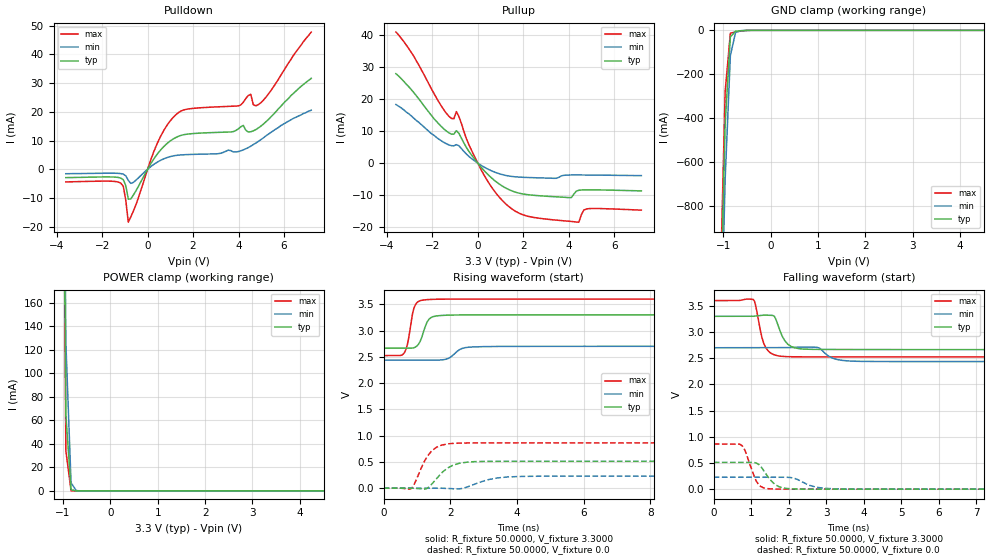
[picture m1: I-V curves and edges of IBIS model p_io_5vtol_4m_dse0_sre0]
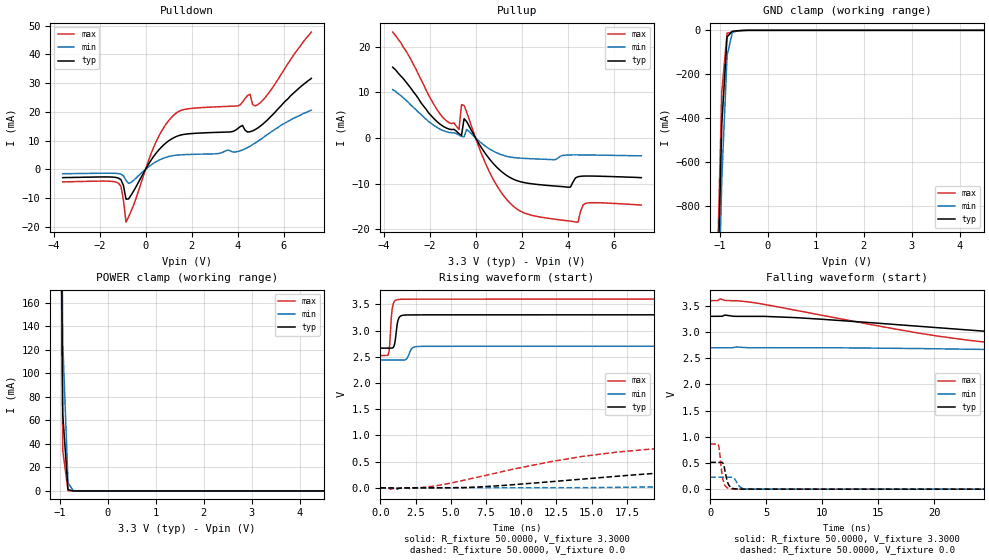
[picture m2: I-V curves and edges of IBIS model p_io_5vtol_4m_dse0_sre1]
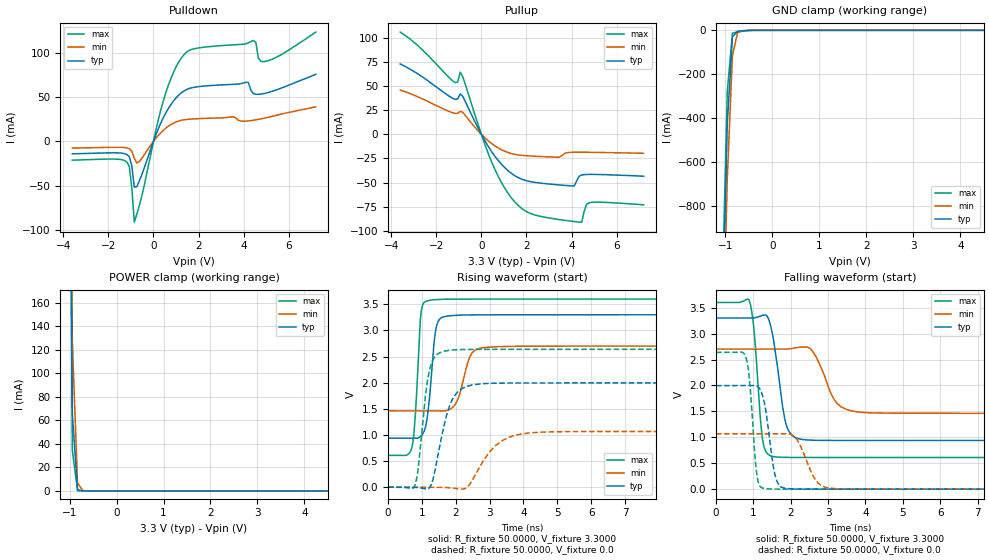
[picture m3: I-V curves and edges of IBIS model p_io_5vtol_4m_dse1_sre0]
| IBIS file nevis_80lqfp_normal.ibs generated by Daphne version: 2018.03.27
[IBIS Ver]   5.0
[Comment Char]   |_char
[File Name]   nevis_80lqfp_normal.ibs
[File Rev]   1
[Date]   Tue Nov  6 16:55:37 2018
[Source]   NXP Viper 2018.03.27
[Notes]
[Disclaimer] IMPORTANT NOTICE
  This information is provided on an AS IS basis and without warranty.
  IN NO EVENT SHALL NXP BE LIABLE FOR INCIDENTAL OR CONSEQUENTIAL
  DAMAGES ARISING FROM USE OF THIS INFORMATION. THIS DISCLAIMER OF
  WARRANTY EXTENDS TO THE USER OF THE INFORMATION, AND TO THEIR CUSTOMERS
  OR USERS OF PRODUCTS  AND IS IN LIEU OF ALL WARRANTIES WHETHER EXPRESS,
  IMPLIED, OR STATUTORY, INCLUDING IMPLIED WARRANTIES OF MERCHANTABILITY
  OR FITNESS FOR PARTICULAR PURPOSE.
  NXP does not represent or warrant that the information furnished
  hereunder is free of infringement of any third party patents,
  copyrights, trade secrets, or other intellectual property rights.
  NXP does not represent or warrant that the information is free of
  defect, or that it meets any particular standard, requirements or need
  of the user of the infomation or their customers.
  NXP reserves the right to change the information in this file
  without notice.
   http://www.nxp.com
[Copyright]   (C) Copyright NXP 2004 - 2018, All Rights Reserved.
|   NEVIS:80LQFP
[Component]   NEVIS:80LQFP
[Manufacturer]   NXP
[Package]
| variable   typ   min   max
R_pkg   0.14792   0.086913   0.16418
L_pkg   3.915e-09   3.208e-09   4.513e-09
C_pkg   6.180e-13   5.453e-13   7.626e-13
[Pin] signal_name   model_name   R_pin   L_pin   C_pin
1   TCK   p_io_5vtol_4m   0.1569   4.463e-09 6.104e-13
2   RESETB   p_vpp_5vtol_4m   0.086913  3.716e-09 7.626e-13
3   GPIOC0   p_io_5vtol_4m   0.1464   4.224e-09 6.498e-13
4   GPIOC1   p_io_5vtol_4m   0.14132   4.089e-09 6.578e-13
5   GPIOC2   p_io_5vtol_4m   0.13836   3.977e-09 6.265e-13
6   GPIOF8   p_io_5vtol_4m   0.13627   3.873e-09 6.056e-13
7   GPIOD6   p_io_5vtol_4m   0.13889   3.853e-09 6.753e-13
8   GPIOD5   p_io_5vtol_4m   0.13733   3.661e-09 5.770e-13
9   GPIOC3   p_io_5vtol_4m   0.13967   3.625e-09 5.687e-13
10   GPIOC4   p_io_5vtol_4m   0.14324   3.260e-09 5.584e-13
11   VSS   GND   NA   NA   NA
12   VDD   POWER   NA   NA   NA
13   GPIOA7   p_io_5vtol_4m   0.14268   3.208e-09 5.596e-13
14   GPIOA6   p_io_5vtol_4m   0.13768   3.627e-09 5.771e-13
15   GPIOA5   p_io_5vtol_4m   0.13834   3.794e-09 6.092e-13
16   GPIOA4   p_io_5vtol_4m   0.14103   3.970e-09 6.163e-13
17   GPIOA0   p_io_5vtol_4m   0.14398   4.103e-09 6.334e-13
18   GPIOA1   p_io_5vtol_4m   0.14886   4.265e-09 6.523e-13
19   GPIOA2   p_io_5vtol_4m   0.15426   4.392e-09 6.811e-13
20   GPIOA3   p_io_5vtol_4m   0.15897   4.513e-09 6.239e-13
21   GPIOB7   p_io_5vtol_4m   0.16119   4.455e-09 6.055e-13
22   GPIOC5   p_io_5vtol_4m   0.089097  3.705e-09 7.594e-13
23   GPIOB6   p_io_5vtol_4m   0.15247   4.133e-09 6.437e-13
24   GPIOB5   p_io_5vtol_4m   0.15127   3.904e-09 6.550e-13
25   GPIOB4   p_io_5vtol_4m   0.15683   3.445e-09 6.248e-13
26   VDDA   POWER   NA   NA   NA
27   VSSA   GND   NA   NA   NA
28   GPIOB0   p_io_5vtol_4m   0.15671   3.227e-09 5.981e-13
29   GPIOB1   p_io_5vtol_4m   0.16081   3.366e-09 5.864e-13
30   VDD   POWER   NA   NA   NA
31   GPIOB2   p_io_5vtol_4m   0.16418   3.339e-09 5.839e-13
32   GPIOA11   p_io_5vtol_4m   0.15928   3.765e-09 5.648e-13
33   GPIOB8   p_io_5vtol_4m   0.15865   3.789e-09 5.728e-13
34   GPIOB3   p_io_5vtol_4m   0.15776   3.412e-09 5.725e-13
35   VDD33   POWER   NA   NA   NA
36   VSS   GND   NA   NA   NA
37   GPIOD7   p_io_5vtol_4m   0.15661   3.718e-09 6.186e-13
38   GPIOG11   p_io_5vtol_4m   0.15508   4.092e-09 6.428e-13
39   GPIOC6   p_io_5vtol_4m   0.15749   4.282e-09 6.708e-13
40   GPIOC7   p_io_5vtol_4m   0.16015   4.420e-09 6.086e-13
41   GPIOC8   p_io_5vtol_4m   0.155   4.392e-09 6.129e-13
42   GPIOC9   p_io_5vtol_4m   0.15023   4.314e-09 6.746e-13
43   GPIOC10   p_io_5vtol_4m   0.14475   4.157e-09 6.325e-13
44   GPIOF0   p_io_5vtol_4m   0.14034   4.038e-09 6.186e-13
45   GPIOF10   p_io_5vtol_4m   0.13729   3.935e-09 5.995e-13
46   GPIOF9   p_io_5vtol_4m   0.13506   3.812e-09 5.800e-13
47   GPIOC11   p_io_5vtol_4m   0.13569   3.773e-09 5.736e-13
48   GPIOC12   p_io_5vtol_4m   0.13431   3.631e-09 5.670e-13
49   GPIOF2   p_io_5vtol_4m   0.13671   3.678e-09 5.521e-13
50   GPIOF3   p_io_5vtol_4m   0.13715   3.575e-09 5.842e-13
51   GPIOF4   p_io_5vtol_4m   0.13922   3.499e-09 5.749e-13
52   GPIOF5   p_io_5vtol_4m   0.14513   3.371e-09 5.453e-13
53   VSS   GND   NA   NA   NA
54   VDD33   POWER   NA   NA   NA
55   GPIOE0   p_io_5vtol_4m   0.14382   3.257e-09 5.801e-13
56   GPIOE1   p_io_5vtol_4m   0.14278   3.728e-09 6.043e-13
57   GPIOG2   p_io_5vtol_4m   0.14594   4.015e-09 5.873e-13
58   GPIOG3   p_io_5vtol_4m   NA   NA   NA
59   GPIOE2   p_io_5vtol_4m   0.15025   4.275e-09 6.580e-13
60   GPIOE3   p_io_5vtol_4m   0.15495   4.361e-09 6.103e-13
61   GPIOC13   p_io_5vtol_4m   0.15782   4.510e-09 6.206e-13
62   GPIOF1   p_io_5vtol_4m   0.15552   4.467e-09 6.836e-13
63   GPIOG0   p_io_5vtol_4m   0.15239   4.349e-09 6.443e-13
64   GPIOG1   p_io_5vtol_4m   0.15   4.246e-09 6.251e-13
65   GPIOE4   p_io_5vtol_4m   0.15123   4.216e-09 6.160e-13
66   GPIOE5   p_io_5vtol_4m   0.14973   4.115e-09 6.183e-13
67   GPIOE6   p_io_5vtol_4m   0.1495   4.063e-09 6.138e-13
68   GPIOE7   p_io_5vtol_4m   0.14975   3.950e-09 6.053e-13
69   GPIOG6   p_io_5vtol_4m   0.15342   4.029e-09 5.810e-13
70   GPIOC14   p_io_5vtol_4m   0.15484   3.948e-09 6.094e-13
71   GPIOC15   p_io_5vtol_4m   0.15791   3.901e-09 6.007e-13
72   GPIOG7   p_io_5vtol_4m   0.16357   3.560e-09 5.812e-13
73   VDD   POWER   NA   NA   NA
74   GPIOF6   p_io_5vtol_4m   0.16081   3.496e-09 6.833e-13
75   GPIOF7   p_io_5vtol_4m   0.16138   3.528e-09 6.113e-13
76   VDD33   POWER   NA   NA   NA
77   VSS   GND   NA   NA   NA
78   TDO   p_io_5vtol_4m   0.16287   3.741e-09 6.499e-13
79   TMS   p_io_5vtol_4m   0.16067   4.282e-09 7.221e-13
80   TDI   p_io_5vtol_4m   0.16215   4.444e-09 6.324e-13
81   NC   NC   NA   NA   NA
[Pin Mapping]   pulldown_ref   pullup_ref
1   NC   NC
2   NC   NC
3   NC   NC
4   NC   NC
5   NC   NC
6   NC   NC
7   NC   NC
8   NC   NC
9   NC   NC
10   NC   NC
11   VSS   NC
12   NC   VDD
13   NC   NC
14   NC   NC
15   NC   NC
16   NC   NC
17   NC   NC
18   NC   NC
19   NC   NC
20   NC   NC
21   NC   NC
22   NC   NC
23   NC   NC
24   NC   NC
25   NC   NC
26   NC   VDDA
27   VSSA   NC
28   NC   NC
29   NC   NC
30   NC   VDD
31   NC   NC
32   NC   NC
33   NC   NC
34   NC   NC
35   NC   VDD33
36   VSS   NC
37   NC   NC
38   NC   NC
39   NC   NC
40   NC   NC
41   NC   NC
42   NC   NC
43   NC   NC
44   NC   NC
45   NC   NC
46   NC   NC
47   NC   NC
48   NC   NC
49   NC   NC
50   NC   NC
51   NC   NC
52   NC   NC
53   VSS   NC
54   NC   VDD33
55   NC   NC
56   NC   NC
57   NC   NC
58   NC   NC
59   NC   NC
60   NC   NC
61   NC   NC
62   NC   NC
63   NC   NC
64   NC   NC
65   NC   NC
66   NC   NC
67   NC   NC
68   NC   NC
69   NC   NC
70   NC   NC
71   NC   NC
72   NC   NC
73   NC   VDD
74   NC   NC
75   NC   NC
76   NC   VDD33
77   VSS   NC
78   NC   NC
79   NC   NC
80   NC   NC
81   NC   NC
|*   Model Selector   *
[Model Selector] p_io_5vtol_4m
p_io_5vtol_4m_dse1_sre0   io, full drive mode without slew rate
p_io_5vtol_4m_dse1_sre1   io, full drive mode with slew rate
p_io_5vtol_4m_dse0_sre0   io, low drive mode without slew rate
p_io_5vtol_4m_dse0_sre1   io, low drive mode with slew rate
| End [Component] NEVIS:80LQFP
| Models and submodels in the file (5): p_io_5vtol_4m_dse0_sre0 (I/O), p_io_5vtol_4m_dse0_sre1 (I/O), p_io_5vtol_4m_dse1_sre0 (I/O), p_io_5vtol_4m_dse1_sre1 (I/O), p_vpp_5vtol_4m (I/O_open_drain)
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[Model] p_io_5vtol_4m_dse0_sre0
|   Model p_io_5vtol_4m_dse0_sre0
| Library cells for typ/min/max conditions are connected as defined below:
|  pad - External Pad
|  ipp_do - Core Input
|  ipp_obe - Output Buffer Enable
|  esd_boost - vdd_s_3v
|  esd_bus - vdd_s_3v
|  ipp_ame - vss_s_lv
|  ipp_dse - vss_s_lv
|  ipp_ina40a_5vtol - NC
|  ipp_ina40b_5vtol - NC
|  ipp_ina_5vtol - NC
|  ipp_ina_mux_3v - NC
|  ipp_ind - NC
|  ipp_ind_3v - NC
|  ipp_pue - vss_s_lv
|  ipp_sre - vss_s_lv
|  tie_3v - vdd_s_3v
|  tie_hi - vdd_s_lv
|  vbuf_3v - vdd_s_3v
|  vdd_bulk_lv - vdd_s_lv
|  vdd_s_3v - vdd_s_3v
|  vdd_s_lv - vdd_s_lv
|  vss_bulk - vss_s_3v
|  vss_s_3v - vss_s_3v
|  vss_s_lv - vss_s_lv
| All other pins connected to ground
Model_type I/O
Polarity   Non-Inverting
Enable   Active-High
Vinl =   1.1550V
Vinh =   2.3100V
Vmeas =  1.6500V
Cref =   25.0000pF
Rref =   0.5000k
Vref =   0.0V
C_comp   2.7442pF   2.6088pF   2.9166pF
[Temperature Range]   25.0000   0.1250k   -40.0000
[Voltage Range]   3.3000V   2.7000V   3.6000V
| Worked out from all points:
|   slope of the pulldown table from 0 to 0.495 V, typ, clamps not added: 82.8 ohm
|   slope of the pullup table from 0 to 0.495 V, typ, clamps not added: 127 ohm
|   GND clamp passes 1 mA (typ) near -0.56 V on its own axis
|   POWER clamp passes 1 mA (typ) near -0.82 V on its own axis
|   rising waveform, R_fixture 50.0000, V_fixture 3.3000: 20-80 % time 220ps typ, 318ps min, 177ps max; typ from 2.66 V to 3.3 V
|   rising waveform, R_fixture 50.0000, V_fixture 0.0: 20-80 % time 520ps typ, 708ps min, 427ps max; typ from 0 V to 0.512 V
|   falling waveform, R_fixture 50.0000, V_fixture 3.3000: 20-80 % time 253ps typ, 333ps min, 210ps max; typ from 3.3 V to 2.66 V
|   falling waveform, R_fixture 50.0000, V_fixture 0.0: 20-80 % time 337ps typ, 455ps min, 264ps max; typ from 0.512 V to 0 V
[Pulldown]
|Voltage   I(typ)   I(min)   I(max)
-3.6V     -2.92mA    -1.56mA    -4.41mA
-1.18V    -3.075mA   -1.514mA   -4.85mA
-1.07V    -3.642mA   -1.711mA   -5.917mA
-850mV    -10.41mA   -3.881mA   -18.45mA
360mV     4.579mA    2.156mA    7.833mA
1.13V     10.56mA    4.658mA    18.11mA
1.79V     12.28mA    5.123mA    21mA
3.99V     14.08mA    6.16mA     22.06mA
4.54V     13.07mA    8.03mA     26.11mA
4.65V     13.38mA    8.6mA      22.52mA
4.87V     14.37mA    9.7mA      22.49mA
7.2V      31.7mA     20.6mA     47.8mA
[Pullup]
|Voltage   I(typ)   I(min)   I(max)
-3.6V     27.9mA     18.3mA     40.9mA
-2.81V    22mA       14mA       33.3mA
-1.38V    10.01mA    6.04mA     15.54mA
-1.05V    9.045mA    5.403mA    13.85mA
-940mV    10.12mA    5.768mA    16.08mA
-390mV    3.678mA    2.088mA    5.744mA
270mV     -2.258mA   -1.197mA   -3.638mA
1.48V     -8.613mA   -4.152mA   -14.19mA
4.01V     -10.78mA   -3.728mA   -18.16mA
4.45V     -8.487mA   -3.709mA   -18.45mA
4.78V     -8.342mA   -3.73mA    -14.33mA
7.2V      -8.69mA    -3.91mA    -14.69mA
[GND_clamp]
|Voltage   I(typ)   I(min)   I(max)
-3.6V     -31.15A    -31.13A    -31.21A
-1.07V    -1.387A    -1.641A    -1.238A
-960mV    -429.3mA   -680.2mA   -281.1mA
-850mV    -29.75mA   -116.1mA   -13.24mA
-740mV    -4.234mA   -9.703mA   -7.092mA
-630mV    -1.925mA   -1.63mA    -3.569mA
-410mV    -31.96uA   -64.36uA   -35uA
7.2V      0A         0A         0A
[POWER_clamp]
|Voltage   I(typ)   I(min)   I(max)
-3.6V     31.35A     31.03A     31.61A
-1.05V    682.2mA    740.4mA    662.9mA
-940mV    65.1mA     126.6mA    34.32mA
-830mV    1.105mA    6.829mA    165.4uA
-720mV    15.33uA    281.3uA    694.4nA
-610mV    212.1nA    11.41uA    2.964nA
7.2V      0A         0A         0A
[Ramp]
| variable   typ   min   max
dV/dt_r  0.3070/0.5203n   0.1368/0.7078n   0.5174/0.4265n
dV/dt_f  0.3816/0.2526n   0.1581/0.3329n   0.6454/0.2102n
R_load = 50.0000
[Rising Waveform]
R_fixture= 50.0000
V_fixture= 3.3000
V_fixture_min= 2.7000
V_fixture_max= 3.6000
|time   V(typ)   V(min)   V(max)
0s        2.664V     2.436V     2.524V
610.3ps   2.664V     2.436V     2.569V
714.5ps   2.664V     2.436V     2.741V
910.9ps   2.675V     2.436V     3.431V
1.094ns   2.792V     2.437V     3.568V
1.273ns   3.119V     2.437V     3.588V
1.552ns   3.276V     2.437V     3.596V
2.35ns    3.298V     2.659V     3.599V
2.979ns   3.3V       2.694V     3.599V
20ns      3.3V       2.7V       3.6V
[Rising Waveform]
R_fixture= 50.0000
V_fixture= 0.0
V_fixture_min= 0.0
V_fixture_max= 0.0
|time   V(typ)   V(min)   V(max)
0s        1.096nV    96.66nV    914.3pV
817.3ps   -174.2uV   1.791uV    -11.85mV
1.238ns   -20.09mV   132uV      527.3mV
1.432ns   68.46mV    364.3uV    703.1mV
1.774ns   310.6mV    -2.683mV   823mV
2.042ns   424.3mV    -10.1mV    850.1mV
2.694ns   503.4mV    66.34mV    860.8mV
3.192ns   509.9mV    168.5mV    861.5mV
4.049ns   511.3mV    221.6mV    861.7mV
20ns      511.7mV    228.1mV    862.3mV
[Falling Waveform]
R_fixture= 50.0000
V_fixture= 3.3000
V_fixture_min= 2.7000
V_fixture_max= 3.6000
|time   V(typ)   V(min)   V(max)
0s        3.3V       2.7V       3.6V
1.056ns   3.301V     2.7V       3.62V
1.285ns   3.321V     2.7V       2.894V
1.39ns    3.322V     2.7V       2.695V
1.614ns   3.301V     2.7V       2.565V
1.898ns   2.83V      2.7V       2.531V
2.744ns   2.668V     2.71V      2.525V
3.178ns   2.667V     2.499V     2.525V
3.812ns   2.665V     2.441V     2.525V
20ns      2.664V     2.436V     2.524V
[Falling Waveform]
R_fixture= 50.0000
V_fixture= 0.0
V_fixture_min= 0.0
V_fixture_max= 0.0
|time   V(typ)   V(min)   V(max)
0s        511.8mV    228.1mV    862.4mV
740.7ps   511.8mV    228.1mV    838mV
824.6ps   511.7mV    228.1mV    750.7mV
1.166ns   486.7mV    228.1mV    119mV
1.481ns   202.1mV    228.1mV    6.302mV
1.652ns   81.2mV     228mV      2.01mV
1.911ns   16.02mV    227.7mV    767.9uV
2.752ns   448uV      36.41mV    432.9uV
3.473ns   288.4uV    2.353mV    359uV
20ns      60.38uV    38.43uV    87.29uV
[Model] p_io_5vtol_4m_dse0_sre1
|   Model p_io_5vtol_4m_dse0_sre1
| Library cells for typ/min/max conditions are connected as defined below:
|  pad - External Pad
|  ipp_do - Core Input
|  ipp_obe - Output Buffer Enable
|  esd_boost - vdd_s_3v
|  esd_bus - vdd_s_3v
|  ipp_ame - vss_s_lv
|  ipp_dse - vss_s_lv
|  ipp_ina40a_5vtol - NC
|  ipp_ina40b_5vtol - NC
|  ipp_ina_5vtol - NC
|  ipp_ina_mux_3v - NC
|  ipp_ind - NC
|  ipp_ind_3v - NC
|  ipp_pue - vss_s_lv
|  ipp_sre - vdd_s_lv
|  tie_3v - vdd_s_3v
|  tie_hi - vdd_s_lv
|  vbuf_3v - vdd_s_3v
|  vdd_bulk_lv - vdd_s_lv
|  vdd_s_3v - vdd_s_3v
|  vdd_s_lv - vdd_s_lv
|  vss_bulk - vss_s_3v
|  vss_s_3v - vss_s_3v
|  vss_s_lv - vss_s_lv
| All other pins connected to ground
Model_type I/O
Polarity   Non-Inverting
Enable   Active-High
Vinl =   1.1550V
Vinh =   2.3100V
Vmeas =  1.6500V
Cref =   25.0000pF
Rref =   0.5000k
Vref =   0.0V
C_comp   2.7442pF   2.6088pF   2.9166pF
[Temperature Range]   25.0000   0.1250k   -40.0000
[Voltage Range]   3.3000V   2.7000V   3.6000V
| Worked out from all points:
|   slope of the pulldown table from 0 to 0.495 V, typ, clamps not added: 82.8 ohm
|   slope of the pullup table from 0 to 0.495 V, typ, clamps not added: 127 ohm
|   GND clamp passes 1 mA (typ) near -0.56 V on its own axis
|   POWER clamp passes 1 mA (typ) near -0.82 V on its own axis
|   rising waveform, R_fixture 50.0000, V_fixture 3.3000: 20-80 % time 192ps typ, 268ps min, 163ps max; typ from 2.66 V to 3.3 V
|   rising waveform, R_fixture 50.0000, V_fixture 0.0: 20-80 % time 17.3ns typ, 32.4ns min, 10.8ns max; typ from 0 V to 0.512 V
|   falling waveform, R_fixture 50.0000, V_fixture 3.3000: 20-80 % time 29.9ns typ, 51ns min, 19.5ns max; typ from 3.3 V to 2.66 V
|   falling waveform, R_fixture 50.0000, V_fixture 0.0: 20-80 % time 342ps typ, 422ps min, 300ps max; typ from 0.512 V to 0 V
[Pulldown]
|Voltage   I(typ)   I(min)   I(max)
-3.6V     -2.92mA    -1.56mA    -4.41mA
-1.18V    -3.075mA   -1.514mA   -4.85mA
-1.07V    -3.642mA   -1.711mA   -5.917mA
-850mV    -10.41mA   -3.881mA   -18.45mA
360mV     4.579mA    2.156mA    7.833mA
1.13V     10.56mA    4.658mA    18.11mA
1.79V     12.28mA    5.123mA    21mA
3.99V     14.08mA    6.16mA     22.06mA
4.54V     13.07mA    8.03mA     26.11mA
4.65V     13.38mA    8.6mA      22.52mA
4.87V     14.37mA    9.7mA      22.49mA
7.2V      31.7mA     20.6mA     47.8mA
[Pullup]
|Voltage   I(typ)   I(min)   I(max)
-3.6V     15.5mA     10.6mA     23.2mA
-1.38V    2.47mA     1.56mA     4.28mA
-720mV    935.3uA    641.5uA    1.84mA
-610mV    580.7uA    348.6uA    7.293mA
-500mV    4.215mA    257.3uA    7.125mA
-390mV    3.605mA    1.85mA     5.718mA
710mV     -5.257mA   -2.715mA   -8.512mA
1.81V     -9.375mA   -4.366mA   -15.61mA
4.12V     -10.77mA   -3.714mA   -18.22mA
4.45V     -8.487mA   -3.709mA   -18.45mA
4.78V     -8.342mA   -3.73mA    -14.33mA
7.2V      -8.69mA    -3.91mA    -14.69mA
[GND_clamp]
|Voltage   I(typ)   I(min)   I(max)
-3.6V     -31.15A    -31.13A    -31.21A
-1.07V    -1.387A    -1.641A    -1.238A
-960mV    -429.3mA   -680.2mA   -281.1mA
-850mV    -29.75mA   -116.1mA   -13.24mA
-740mV    -4.234mA   -9.703mA   -7.092mA
-630mV    -1.925mA   -1.63mA    -3.569mA
-410mV    -31.96uA   -64.36uA   -35uA
7.2V      0A         0A         0A
[POWER_clamp]
|Voltage   I(typ)   I(min)   I(max)
-3.6V     31.35A     31.03A     31.61A
-1.05V    682.2mA    740.4mA    662.9mA
-940mV    65.1mA     126.6mA    34.32mA
-830mV    1.105mA    6.829mA    165.4uA
-720mV    15.33uA    281.3uA    694.4nA
-610mV    212.1nA    11.41uA    2.964nA
7.2V      0A         0A         0A
[Ramp]
| variable   typ   min   max
dV/dt_r  0.3071/17.2926n   0.1369/32.3674n   0.5175/10.7611n
dV/dt_f  0.3817/29.8719n   0.1576/51.0200n   0.6456/19.5314n
R_load = 50.0000
[Rising Waveform]
R_fixture= 50.0000
V_fixture= 3.3000
V_fixture_min= 2.7000
V_fixture_max= 3.6000
|time   V(typ)   V(min)   V(max)
0s        2.664V     2.437V     2.524V
605.3ps   2.664V     2.437V     2.579V
657.9ps   2.664V     2.437V     2.693V
807.7ps   2.664V     2.437V     3.325V
923.6ps   2.679V     2.436V     3.511V
1.276ns   3.209V     2.437V     3.592V
1.646ns   3.293V     2.437V     3.597V
2.341ns   3.298V     2.679V     3.598V
3.739ns   3.299V     2.699V     3.598V
250ns     3.3V       2.7V       3.6V
[Rising Waveform]
R_fixture= 50.0000
V_fixture= 0.0
V_fixture_min= 0.0
V_fixture_max= 0.0
|time   V(typ)   V(min)   V(max)
0s        1.096nV    96.66nV    914.3pV
730.2ps   540.1uV    1.417uV    -25.29mV
3.533ns   -267.8uV   -118.1uV   22.43mV
11.84ns   111.3mV    1.042mV    487mV
16.8ns    222mV      9.094mV    681.3mV
24.08ns   354mV      38.46mV    807.6mV
31.02ns   430.3mV    75.05mV    845.8mV
49.75ns   501.2mV    160.4mV    861.8mV
86.96ns   511.7mV    219.4mV    862.5mV
250ns     511.8mV    228.1mV    862.5mV
[Falling Waveform]
R_fixture= 50.0000
V_fixture= 3.3000
V_fixture_min= 2.7000
V_fixture_max= 3.6000
|time   V(typ)   V(min)   V(max)
0s        3.3V       2.7V       3.6V
896.8ps   3.3V       2.7V       3.63V
3.769ns   3.3V       2.7V       3.565V
18.49ns   3.112V     2.686V     2.984V
25.66ns   2.998V     2.664V     2.78V
33.75ns   2.887V     2.635V     2.66V
43.81ns   2.796V     2.595V     2.594V
65.21ns   2.714V     2.521V     2.543V
96.83ns   2.677V     2.472V     2.527V
250ns     2.664V     2.437V     2.524V
[Falling Waveform]
R_fixture= 50.0000
V_fixture= 0.0
V_fixture_min= 0.0
V_fixture_max= 0.0
|time   V(typ)   V(min)   V(max)
0s        511.8mV    228.1mV    862.4mV
711.3ps   511.8mV    228.1mV    851.3mV
813.8ps   511.8mV    228.1mV    743.1mV
1.045ns   511.3mV    228.1mV    281.6mV
1.18ns    474mV      228.1mV    137.9mV
1.57ns    116.7mV    228mV      19.01mV
2.147ns   7.963mV    204.4mV    2.261mV
2.747ns   1.249mV    29.86mV    1.357mV
3.983ns   641.3uV    486.1uV    1mV
250ns     26.94nV    927.1nV    8.795nV
[Model] p_io_5vtol_4m_dse1_sre0
|   Model p_io_5vtol_4m_dse1_sre0
| Library cells for typ/min/max conditions are connected as defined below:
|  pad - External Pad
|  ipp_do - Core Input
|  ipp_obe - Output Buffer Enable
|  esd_boost - vdd_s_3v
|  esd_bus - vdd_s_3v
|  ipp_ame - vss_s_lv
|  ipp_dse - vdd_s_lv
|  ipp_ina40a_5vtol - NC
|  ipp_ina40b_5vtol - NC
|  ipp_ina_5vtol - NC
|  ipp_ina_mux_3v - NC
|  ipp_ind - NC
|  ipp_ind_3v - NC
|  ipp_pue - vss_s_lv
|  ipp_sre - vss_s_lv
|  tie_3v - vdd_s_3v
|  tie_hi - vdd_s_lv
|  vbuf_3v - vdd_s_3v
|  vdd_bulk_lv - vdd_s_lv
|  vdd_s_3v - vdd_s_3v
|  vdd_s_lv - vdd_s_lv
|  vss_bulk - vss_s_3v
|  vss_s_3v - vss_s_3v
|  vss_s_lv - vss_s_lv
| All other pins connected to ground
Model_type I/O
Polarity   Non-Inverting
Enable   Active-High
Vinl =   1.1550V
Vinh =   2.3100V
Vmeas =  1.6500V
Cref =   25.0000pF
Rref =   0.5000k
Vref =   0.0V
C_comp   2.7442pF   2.6088pF   2.9166pF
[Temperature Range]   25.0000   0.1250k   -40.0000
[Voltage Range]   3.3000V   2.7000V   3.6000V
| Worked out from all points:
|   slope of the pulldown table from 0 to 0.495 V, typ, clamps not added: 16.7 ohm
|   slope of the pullup table from 0 to 0.495 V, typ, clamps not added: 25.7 ohm
|   GND clamp passes 1 mA (typ) near -0.56 V on its own axis
|   POWER clamp passes 1 mA (typ) near -0.82 V on its own axis
|   rising waveform, R_fixture 50.0000, V_fixture 3.3000: 20-80 % time 198ps typ, 316ps min, 148ps max; typ from 0.938 V to 3.3 V
|   rising waveform, R_fixture 50.0000, V_fixture 0.0: 20-80 % time 433ps typ, 731ps min, 266ps max; typ from 0 V to 2 V
|   falling waveform, R_fixture 50.0000, V_fixture 3.3000: 20-80 % time 273ps typ, 438ps min, 181ps max; typ from 3.3 V to 0.939 V
|   falling waveform, R_fixture 50.0000, V_fixture 0.0: 20-80 % time 233ps typ, 387ps min, 161ps max; typ from 2 V to 0 V
[Pulldown]
|Voltage   I(typ)   I(min)   I(max)
-3.6V     -13.95mA   -7.44mA    -21.1mA
-1.18V    -14.7mA    -7.219mA   -23.24mA
-1.07V    -17.36mA   -8.141mA   -28.3mA
-850mV    -51.45mA   -18.95mA   -91.09mA
-630mV    -44.71mA   -22.71mA   -72.44mA
470mV     28.45mA    13.31mA    48.59mA
1.35V     56.89mA    24.4mA     97.86mA
4.1V      66.73mA    22.95mA    110.2mA
4.43V     54.09mA    23.92mA    113.9mA
4.65V     53.15mA    25mA       94.51mA
4.98V     54.48mA    26.7mA     90.35mA
7.2V      75.8mA     39.1mA     123.4mA
[Pullup]
|Voltage   I(typ)   I(min)   I(max)
-3.6V     72.9mA     45.9mA     106mA
-1.16V    36.23mA    21.7mA     53.64mA
-1.05V    36.74mA    21.9mA     54.26mA
-940mV    41.85mA    23.77mA    64.43mA
600mV     -22.66mA   -11.88mA   -36.28mA
1.15V     -36.98mA   -18.56mA   -59.89mA
1.81V     -46.62mA   -21.82mA   -77.16mA
4.12V     -53.36mA   -18.54mA   -90.34mA
4.45V     -42.19mA   -18.52mA   -91.04mA
4.67V     -41.57mA   -18.57mA   -72.57mA
4.78V     -41.5mA    -18.6mA    -70.99mA
7.2V      -43.39mA   -19.66mA   -73.06mA
[GND_clamp]
|Voltage   I(typ)   I(min)   I(max)
-3.6V     -31.15A    -31.13A    -31.21A
-1.07V    -1.387A    -1.641A    -1.238A
-960mV    -429.3mA   -680.2mA   -281.1mA
-850mV    -29.75mA   -116.1mA   -13.24mA
-740mV    -4.234mA   -9.703mA   -7.092mA
-630mV    -1.925mA   -1.63mA    -3.569mA
-410mV    -31.96uA   -64.36uA   -35uA
7.2V      0A         0A         0A
[POWER_clamp]
|Voltage   I(typ)   I(min)   I(max)
-3.6V     31.35A     31.03A     31.61A
-1.05V    682.2mA    740.4mA    662.9mA
-940mV    65.1mA     126.6mA    34.32mA
-830mV    1.105mA    6.829mA    165.4uA
-720mV    15.33uA    281.3uA    694.4nA
-610mV    212.1nA    11.41uA    2.964nA
7.2V      0A         0A         0A
[Ramp]
| variable   typ   min   max
dV/dt_r  1.1975/0.4329n   0.6401/0.7312n   1.5830/0.2663n
dV/dt_f  1.4166/0.2733n   0.7428/0.4382n   1.7935/0.1810n
R_load = 50.0000
[Rising Waveform]
R_fixture= 50.0000
V_fixture= 3.3000
V_fixture_min= 2.7000
V_fixture_max= 3.6000
|time   V(typ)   V(min)   V(max)
0s        938.5mV    1.461V     610.4mV
700.1ps   938.2mV    1.461V     747.1mV
796.4ps   936.7mV    1.461V     1.287V
950.6ps   966.3mV    1.461V     3.178V
1.101ns   1.142V     1.462V     3.551V
1.388ns   2.926V     1.461V     3.588V
1.622ns   3.255V     1.459V     3.595V
1.984ns   3.288V     1.584V     3.598V
2.713ns   3.298V     2.658V     3.599V
10ns      3.3V       2.7V       3.6V
[Rising Waveform]
R_fixture= 50.0000
V_fixture= 0.0
V_fixture_min= 0.0
V_fixture_max= 0.0
|time   V(typ)   V(min)   V(max)
0s        411.9pV    47.82nV    286.1pV
789.5ps   -503.9uV   655.3nV    31.27mV
878.5ps   -6.744mV   -6.775uV   304.7mV
1.188ns   -27.08mV   110.8uV    2.128V
1.538ns   828.6mV    -14.89uV   2.576V
1.891ns   1.669V     -15.27mV   2.625V
2.523ns   1.961V     173.5mV    2.637V
3.139ns   1.99V      774.3mV    2.638V
3.956ns   1.995V     1.021V     2.638V
10ns      1.996V     1.067V     2.638V
[Falling Waveform]
R_fixture= 50.0000
V_fixture= 3.3000
V_fixture_min= 2.7000
V_fixture_max= 3.6000
|time   V(typ)   V(min)   V(max)
0s        3.3V       2.7V       3.6V
897ps     3.3V       2.7V       3.62V
1.012ns   3.302V     2.7V       3.118V
1.248ns   3.352V     2.7V       952.4mV
1.481ns   3.092V     2.7V       637.9mV
1.861ns   1.291V     2.7V       613mV
2.204ns   973.7mV    2.735V     611.7mV
2.551ns   944.9mV    2.689V     611.3mV
3.583ns   939.7mV    1.518V     611mV
10ns      939mV      1.462V     610.8mV
[Falling Waveform]
R_fixture= 50.0000
V_fixture= 0.0
V_fixture_min= 0.0
V_fixture_max= 0.0
|time   V(typ)   V(min)   V(max)
0s        1.996V     1.067V     2.639V
793.2ps   1.996V     1.067V     2.557V
892.4ps   1.996V     1.067V     2.131V
1.088ns   1.992V     1.067V     303.9mV
1.245ns   1.808V     1.067V     21.49mV
1.576ns   285.6mV    1.067V     1.916mV
1.813ns   22.93mV    1.069V     779.9uV
2.113ns   4.177mV    1.006V     534.5uV
2.932ns   535.4uV    34.39mV    380.9uV
10ns      242.2uV    204.3uV    218.8uV
